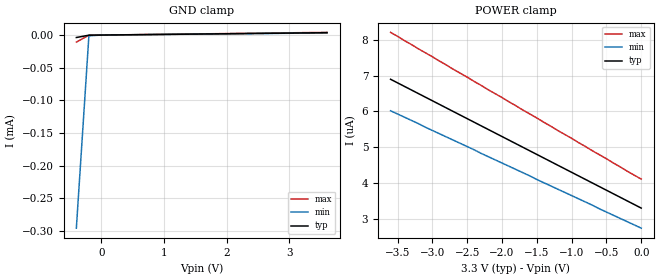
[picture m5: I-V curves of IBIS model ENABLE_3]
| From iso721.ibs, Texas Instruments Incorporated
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|   Output Enable 3.3V
[Model]   ENABLE_3
Model_type   Input
|Signals   EN
Vinh = 2.0
Vinl = 0.8
|   typ   min   max
C_comp   1.3pF   1.1pF   1.5pF
|   typ   min   max
[Temperature Range]   27   -40   125
[Voltage range]   3.3V   3.0V   3.6V
[GND_clamp]
|   Voltage   I(typ)   I(min)   I(max)
-400mV    -3.79uA    -296uA     -10.8uA
-200mV    -202nA     -1.2uA     -230nA
0V        0A         0A         0A
3.6V      3.6uA      3.28uA     4.11uA
[Power_clamp]
| Note that the[POWER_clamp]voltage table is referenced to Vcc
| and is calculated using Vtable=Vcc - Vmeasured.
|   Voltage   I(typ)   I(min)   I(max)
-3.6V     6.9uA      6.02uA     8.21uA
-500mV    3.8uA      3.19uA     4.68uA
-200mV    3.5uA      2.92uA     4.33uA
0V        3.3uA      2.74uA     4.11uA
